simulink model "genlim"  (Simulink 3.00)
settings: Solver=ode45  StartTime=0.0  StopTime=10  RelTol=1e-6  AbsTol=1e-6

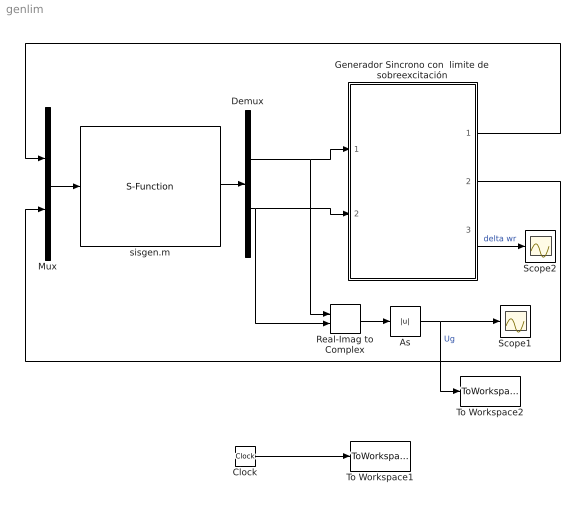
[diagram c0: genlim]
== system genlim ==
  As : Abs
  Clock : Clock
  Demux : Demux  Outputs=2
  Generador Sincrono con  limite de sobreexcitación : Subsystem  mask{Ug=1.0165, teta=8.8871, Pg=1.094, Qg=0.0165, Xd=1.31875, Xq=1.2625, Xdp=0.175, Ra=0.002875, H=3.712, Emin=-5.73, Emax=5.73, Tdp=4.2, K=200, K1=100, K2=1/12, A=1, Ifdlimit=2.17}
      mask prompts: Ug "Módulo de la tensión de alimentación [ pu. ]"; teta "Fase de la tensión de alimentación [ ° ]"; Pg "Potencia activa generada inicial [ pu. ]"; Qg "Potencia reactiva generada inicial  [ pu. ]"; Xd "Reactancia Síncrona  de Eje d ,  Xd  (p.u.)"; Xq "Reactancia Síncrona  de Eje q,  Xq  (p.u.)"; Xdp "Reactancia Subtransitoria de eje d,  X'd  (p.u.)"; Ra "Resistencia de Estator,  Ra  (p.u.)"; H "Constante de Inercia H (s)"; Emin "Limite Inferior Regulador de Tensión,  Efmin"; Emax "Límite Superior Regulador, Efmax"; Tdp "Constante de Tiempo del Rotor T'd (s)"; K "Ganancia del Regulador de tensión K"; K1 "Constante K1 de la sobreexcitación"; K2 "Constante K2 de la sobreexcitación"; A "Límite máximo de la sobreexcitación, A"; Ifdlimit "Límite de la corriente de campo , Ifd limit"
  Mux : Mux  Inputs=2
  Real-Imag to Complex : RealImagToComplex  Input=RealAndImag  ConstantPart=0
  Scope1 : Scope
  Scope2 : Scope
  To Workspace1 : ToWorkspace  VariableName=t  SampleTime=-1  SaveFormat=Matrix
  To Workspace2 : ToWorkspace  VariableName=U  SampleTime=-1  SaveFormat=Matrix
  sisgen.m : S-Function  FunctionName=sisgen  Parameters=U1,teta,Rsis,Xsis  PortCounts=[]  SFunctionModules=''  mask{U1=1.0788, teta=5.0972, Rsis=0, Xsis=0.0625}
      mask prompts: U1 "Módulo de la tensión del sistema [ pu. ]"; teta "Fase de la tensión del Sistema [ ° ]"; Rsis "Resistencia del sistema equivalente [ pu. ]"; Xsis "Reactancia del sistema equivalente"
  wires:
  sisgen.m/1 -> Demux/1
  Demux/2 -> Generador Sincrono con  limite de sobreexcitación/2(Ugimag), Real-Imag to Complex/2
  Mux/1 -> sisgen.m/1
  Demux/1 -> Generador Sincrono con  limite de sobreexcitación/1(Ugreal), Real-Imag to Complex/1
  Generador Sincrono con  limite de sobreexcitación/3(Delta Wr) -> Scope2/1  "delta wr"
  Generador Sincrono con  limite de sobreexcitación/1(Igreal) -> Mux/1
  Generador Sincrono con  limite de sobreexcitación/2(Igimag) -> Mux/2
  Real-Imag to Complex/1 -> As/1
  Clock/1 -> To Workspace1/1
  As/1 -> Scope1/1, To Workspace2/1  "Ug"

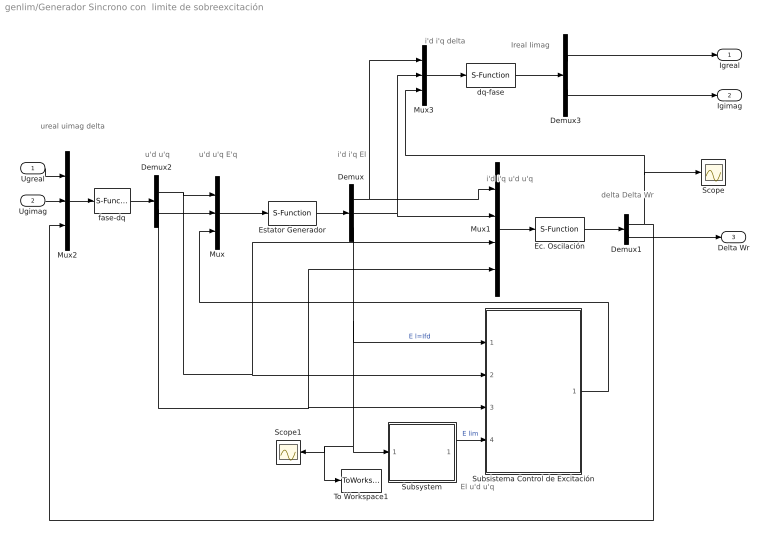
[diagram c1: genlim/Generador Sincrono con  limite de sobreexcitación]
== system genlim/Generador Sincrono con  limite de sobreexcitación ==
  note: u'd u'q E'q
  note: i'd i'q El
  note: i'd i'q u'd u'q
  note: delta Delta Wr
  note: El u'd u'q
  note: ureal uimag delta
  note: u'd u'q
  note: i'd i'q delta
  note: Ireal Iimag
  Ugreal : Inport  Port=1  PortWidth=-1  SampleTime=-1  DataType=auto
  Ugimag : Inport  Port=2  PortWidth=-1  SampleTime=-1  DataType=auto
  Demux : Demux  Outputs=3
  Demux1 : Demux  Outputs=2
  Demux2 : Demux  Outputs=2
  Demux3 : Demux  Outputs=2
  Ec. Oscilación : S-Function  FunctionName=genosc  Parameters=H,Ug,teta,Pg,Qg,Ra,Xd,Xq,Xdp,K  PortCounts=[]  SFunctionModules=''
  Estator Generador : S-Function  FunctionName=gsinc2  Parameters=Ra, Xd, Xq, Xdp  PortCounts=[]  SFunctionModules=''
  Mux : Mux  Inputs=3
  Mux1 : Mux  Inputs=4
  Mux2 : Mux  Inputs=3
  Mux3 : Mux  Inputs=3
  Scope : Scope
  Scope1 : Scope
  Subsistema Control de Excitación : Subsystem  mask{Tdp=Tdp, Emax=Emax, Emin=Emin, K=K}
      mask prompts: Tdp "Cte. Tiempo Rotor"; K "Ganancia Regulador"
  Subsystem : Subsystem  mask{Ifdlimit=Ifdlimit, K2=K2, K1=K1, A=A}
      mask prompts: Ifdlimit "Límite máximo de la corriente de campo  [ pu. ]"; K2 "Cosntante K2"; K1 "Constante K1"; A "Límite Superior de la sobreexcitación .  A"
  To Workspace1 : ToWorkspace  VariableName=El  SampleTime=-1  SaveFormat=Matrix
  dq-fase : S-Function  FunctionName=Tdqf  PortCounts=[]  SFunctionModules=''
  fase-dq : S-Function  FunctionName=Tfdq  PortCounts=[]  SFunctionModules=''
  Igreal : Outport  Port=1
  Igimag : Outport  Port=2
  Delta Wr : Outport  Port=3
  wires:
  Estator Generador/1 -> Demux/1
  Mux3/1 -> dq-fase/1
  dq-fase/1 -> Demux3/1
  Demux3/1 -> Igreal/1
  Demux3/2 -> Igimag/1
  Mux2/1 -> fase-dq/1
  Ugreal/1 -> Mux2/1
  Ugimag/1 -> Mux2/2
  fase-dq/1 -> Demux2/1
  Demux2/1 -> Mux/1, Subsistema Control de Excitación/2(u'd), Mux1/3
  Demux2/2 -> Mux/2, Subsistema Control de Excitación/3(u'q), Mux1/4
  Mux/1 -> Estator Generador/1
  Subsistema Control de Excitación/1(E'q) -> Mux/3
  Mux1/1 -> Ec. Oscilación/1
  Ec. Oscilación/1 -> Demux1/1
  Demux1/2 -> Delta Wr/1
  Demux1/1 -> Mux2/3, Mux3/3, Scope/1
  Demux/1 -> Mux1/1, Mux3/1
  Demux/2 -> Mux1/2, Mux3/2
  Subsystem/1(Elim) -> Subsistema Control de Excitación/4(E lim)  "E lim"
  Demux/3 -> Subsistema Control de Excitación/1(E l), Subsystem/1(Ifd), Scope1/1, To Workspace1/1  "E l=Ifd"

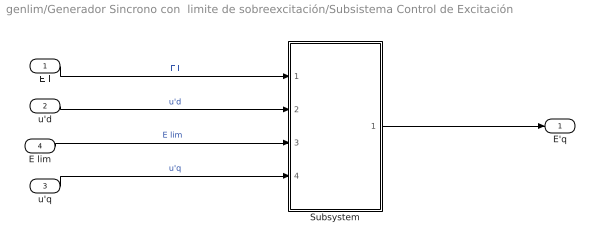
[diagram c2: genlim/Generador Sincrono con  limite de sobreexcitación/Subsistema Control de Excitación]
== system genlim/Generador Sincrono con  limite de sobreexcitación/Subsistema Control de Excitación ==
  E l : Inport  Port=1  PortWidth=-1  SampleTime=-1  DataType=auto
  u'd : Inport  Port=2  PortWidth=-1  SampleTime=-1  DataType=auto
  u'q : Inport  Port=3  PortWidth=-1  SampleTime=-1  DataType=auto
  E lim : Inport  Port=4  PortWidth=-1  SampleTime=-1  DataType=auto
  Subsystem : Subsystem
  E'q : Outport  Port=1
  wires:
  u'd/1 -> Subsystem/2(In2)  "u'd"
  u'q/1 -> Subsystem/4(In4)  "u'q"
  E l/1 -> Subsystem/1(In1)  "E l"
  Subsystem/1(Out1) -> E'q/1
  E lim/1 -> Subsystem/3(In3)  "E lim"

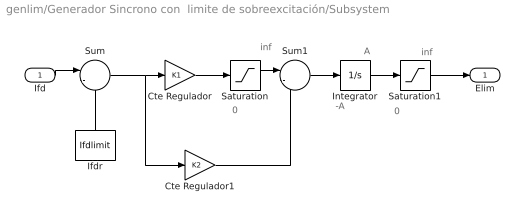
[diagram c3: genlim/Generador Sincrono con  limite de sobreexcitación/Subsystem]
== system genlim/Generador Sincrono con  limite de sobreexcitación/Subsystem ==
  note: -A
  note: A
  note: 0
  note: inf
  note: 0
  note: inf
  Ifd : Inport  Port=1  PortWidth=-1  SampleTime=-1  DataType=auto
  Cte Regulador : Gain  Gain=K1  SaturateOnIntegerOverflow=on
  Cte Regulador1 : Gain  Gain=K2  SaturateOnIntegerOverflow=on
  Ifdr : Constant  Orientation=up  Value=Ifdlimit
  Integrator : Integrator  ExternalReset=none  InitialConditionSource=internal  InitialCondition=-A  LimitOutput=on  UpperSaturationLimit=A  LowerSaturationLimit=-A  ShowSaturationPort=off  ShowStatePort=off  AbsoluteTolerance=auto
  Saturation : Saturate  UpperLimit=10000  LowerLimit=0
  Saturation1 : Saturate  UpperLimit=10000  LowerLimit=0
  Sum : Sum  Inputs=|-+  SaturateOnIntegerOverflow=on
  Sum1 : Sum  Inputs=|--  SaturateOnIntegerOverflow=on
  Elim : Outport  Port=1
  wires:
  Cte Regulador/1 -> Saturation/1
  Saturation/1 -> Sum1/1
  Cte Regulador1/1 -> Sum1/2
  Sum1/1 -> Integrator/1
  Integrator/1 -> Saturation1/1
  Saturation1/1 -> Elim/1
  Sum/1 -> Cte Regulador/1, Cte Regulador1/1
  Ifdr/1 -> Sum/2
  Ifd/1 -> Sum/1

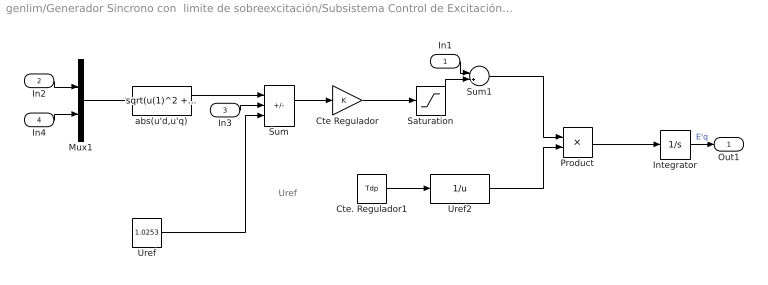
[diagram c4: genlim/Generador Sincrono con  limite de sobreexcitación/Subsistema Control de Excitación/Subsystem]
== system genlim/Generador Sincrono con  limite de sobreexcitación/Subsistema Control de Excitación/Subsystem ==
  note: Uref
  In1 : Inport  Port=1  PortWidth=-1  SampleTime=-1  DataType=auto
  In2 : Inport  Port=2  PortWidth=-1  SampleTime=-1  DataType=auto
  In3 : Inport  Port=3  PortWidth=-1  SampleTime=-1  DataType=auto
  In4 : Inport  Port=4  PortWidth=-1  SampleTime=-1  DataType=auto
  Cte Regulador : Gain  Gain=K  SaturateOnIntegerOverflow=on
  Cte. Regulador1 : Constant  Value=Tdp
  Integrator : Integrator  ExternalReset=none  InitialConditionSource=internal  InitialCondition=0.7710  LimitOutput=off  UpperSaturationLimit=inf  LowerSaturationLimit=-inf  ShowSaturationPort=off  ShowStatePort=off  AbsoluteTolerance=auto
  Mux1 : Mux  Inputs=2
  Product : Product  Inputs=2  SaturateOnIntegerOverflow=on
  Saturation : Saturate  UpperLimit=Emax  LowerLimit=Emin
  Sum : Sum  Inputs=|--+  SaturateOnIntegerOverflow=on
  Sum1 : Sum  Inputs=-+  SaturateOnIntegerOverflow=on
  Uref : Constant  Value=1.0253
  Uref2 : Fcn  Expr=1/u
  abs(u'd,u'q) : Fcn  Expr=sqrt(u(1)^2 + u(2) ^2)
  Out1 : Outport  Port=1
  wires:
  Sum/1 -> Cte Regulador/1
  Cte Regulador/1 -> Saturation/1
  Saturation/1 -> Sum1/2
  Mux1/1 -> abs(u'd,u'q)/1
  abs(u'd,u'q)/1 -> Sum/1
  Cte. Regulador1/1 -> Uref2/1
  Sum1/1 -> Product/1
  Uref2/1 -> Product/2
  Product/1 -> Integrator/1
  Uref/1 -> Sum/3
  In1/1 -> Sum1/1
  In2/1 -> Mux1/1
  In3/1 -> Sum/2
  In4/1 -> Mux1/2
  Integrator/1 -> Out1/1  "E'q"
